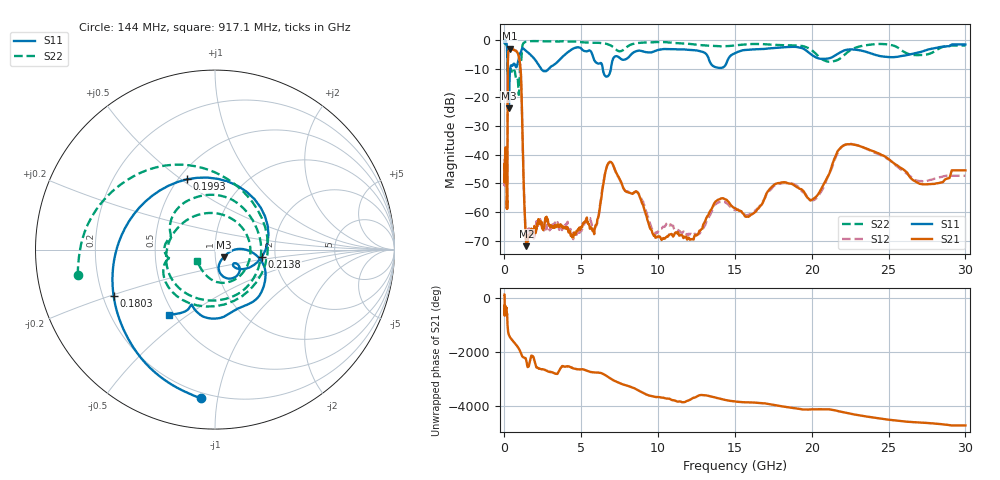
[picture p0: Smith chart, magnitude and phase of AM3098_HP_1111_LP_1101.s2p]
! Date/Time: Thu, Feb 28, 2019 8:48 AM
! Network Analyzer: Agilent Technologies E8364B Rev: A.07.50.67
! Sweep from 0.010 to 30.000 GHz, 1601 Points, Sweep Type: LOG
! Power Supply: 5.023 V, 0.002 A
# Hz S DB R 50
!freq MagS11 AngS11 MagS21 AngS21 MagS12 AngS12 MagS22 AngS22
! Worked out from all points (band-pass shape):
!   1601 points, 10 MHz to 30 GHz, reference 50 ohm
!   highest |S21| = -3.12 dB at 337.1 MHz (marker M1); lowest = -71.8 dB at 1.432 GHz (marker M2)
!   |S21| within 3 dB of the highest: 228.3 MHz to 945.6 MHz (717.3 MHz wide, 122 % of centre)
!   lowest |S11| = -23.9 dB at 293 MHz (marker M3), VSWR 1.14, Z = 54.9 - j4.65 ohm
!   |S11| at or under -10 dB: 210.1 MHz to 373.8 MHz (163.7 MHz wide, 56.1 % of centre); 2.372 GHz to 2.907 GHz (534.5 MHz wide, 20.2 % of centre); 6.391 GHz to 6.931 GHz (540.2 MHz wide, 8.11 % of centre)
!   |S22| runs from -19.1 to -0.4 dB; largest |S21 - S12| = 0.0085
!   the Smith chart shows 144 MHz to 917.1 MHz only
!   S11 on the Smith chart (normalised r, x): 144 MHz: 0.17, -0.89; 180.3 MHz: 0.24, -0.20; 199.3 MHz: 0.55, +0.53; 213.8 MHz: 1.70, -0.14; 917.1 MHz: 0.47, -0.43
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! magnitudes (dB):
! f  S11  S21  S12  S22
! 10 MHz  -0.4  -44.3  -44.0  -0.6
! 38.04 MHz  -0.2  -41.0  -41.2  -0.8
! 84.71 MHz  -0.6  -38.5  -37.8  -1.3
! 144 MHz  -1.6  -53.4  -55.0  -2.2
! 144.7 MHz  -1.6  -53.6  -55.7  -2.2
! 180.3 MHz  -4.1  -58.8  -55.7  -5.3
! 199.3 MHz  -7.5  -35.4  -34.8  -10.7
! 213.8 MHz  -11.5  -12.8  -12.8  -9.5
! 293 MHz  -23.9  -3.3  -3.3  -11.7
! 337.1 MHz  -12.9  -3.1  -3.1  -11.0
! 550.5 MHz  -8.7  -3.4  -3.3  -11.4
! 917.1 MHz  -7.0  -5.5  -5.4  -18.5
! 1.082 GHz  -4.1  -13.3  -13.3  -7.3
! 1.432 GHz  -3.9  -71.8  -70.2  -0.7
! 2.084 GHz  -7.6  -65.8  -63.1  -0.5
! 4.617 GHz  -2.8  -67.8  -67.3  -0.6
! 6.821 GHz  -12.0  -42.6  -42.7  -1.7
! 7.926 GHz  -6.7  -52.8  -52.7  -2.7
! 12.07 GHz  -3.5  -69.6  -67.7  -1.4
! 20.1 GHz  -5.6  -55.3  -55.9  -4.0
! 22.56 GHz  -3.4  -36.3  -36.2  -3.5
! 30 GHz  -1.6  -45.4  -47.3  -2.0
